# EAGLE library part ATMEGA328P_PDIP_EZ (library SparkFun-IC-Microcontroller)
Keyed ATMEGA328 DIP This is a version of the DIP package with pin 28 clipped to prevent reverse insertion. See regular 328 for product references.
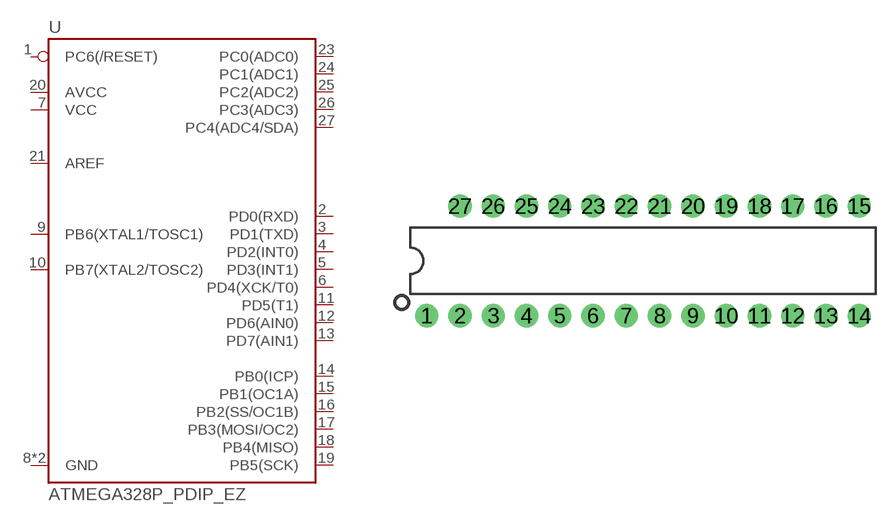
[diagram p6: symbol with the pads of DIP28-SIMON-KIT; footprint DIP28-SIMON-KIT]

Designator prefix U

## ATMEGA328P_PDIP_EZ  [DIP28-SIMON-KIT]
1  PC6(/RESET)
2  PD0(RXD)
3  PD1(TXD)
4  PD2(INT0)
5  PD3(INT1)
6  PD4(XCK/T0)
7  VCC
8  GND
9  PB6(XTAL1/TOSC1)
10  PB7(XTAL2/TOSC2)
11  PD5(T1)
12  PD6(AIN0)
13  PD7(AIN1)
14  PB0(ICP)
15  PB1(OC1A)
16  PB2(SS/OC1B)
17  PB3(MOSI/OC2)
18  PB4(MISO)
19  PB5(SCK)
20  AVCC
21  AREF
22  GND
23  PC0(ADC0)
24  PC1(ADC1)
25  PC2(ADC2)
26  PC3(ADC3)
27  PC4(ADC4/SDA)

## Footprint DIP28-SIMON-KIT (pad centres in mm)
28-pin "EZ" package. Pin 28 is clipped during kitting to key the chip. Pins are spaced a little wider than normal to ease insertion. Top mask deleted so solder can ONLY be applied on bottom.
drill 0.864 pad 1.778: 1 -16.51,-4.191; 2 -13.97,-4.191; 3 -11.43,-4.191; 4 -8.89,-4.191; 5 -6.35,-4.191; 6 -3.81,-4.191; 7 -1.27,-4.191; 8 1.27,-4.191; 9 3.81,-4.191; 10 6.35,-4.191; 11 8.89,-4.191; 12 11.43,-4.191; 13 13.97,-4.191; 14 16.51,-4.191; 15 16.51,4.191; 16 13.97,4.191; 17 11.43,4.191; 18 8.89,4.191; 19 6.35,4.191; 20 3.81,4.191; 21 1.27,4.191; 22 -1.27,4.191; 23 -3.81,4.191; 24 -6.35,4.191; 25 -8.89,4.191; 26 -11.43,4.191; 27 -13.97,4.191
